PROGRAM P_Prog7
VAR

	fbKL6401 		: FB_LON_KL6401;

	fbREAD_191		: FB_READ_191_SNVT_log_status;
	fbSEND_191		: FB_SEND_191_SNVT_log_status;

	fbREAD_192		: FB_READ_192_SNVT_time_stamp_p;
	fbSEND_192		: FB_SEND_192_SNVT_time_stamp_p;

	fbREAD_193		: FB_READ_193_SNVT_log_fx_request;
	fbSEND_193		: FB_SEND_193_SNVT_log_fx_request;

	fbREAD_194		: FB_READ_194_SNVT_log_fx_status;
	fbSEND_194		: FB_SEND_194_SNVT_log_fx_status;

	fbREAD_195		: FB_READ_195_SNVT_log_request;
	fbSEND_195		: FB_SEND_195_SNVT_log_request;

	fbREAD_196		: FB_READ_196_SNVT_enthalpy_d;
	fbSEND_196		: FB_SEND_196_SNVT_enthalpy_d;

	fbREAD_197		: FB_READ_197_SNVT_amp_ac_mil;
	fbSEND_197		: FB_SEND_197_SNVT_amp_ac_mil;

	fbREAD_198		: FB_READ_198_SNVT_time_hour_p;
	fbSEND_198		: FB_SEND_198_SNVT_time_hour_p;

	fbREAD_199		: FB_READ_199_SNVT_lamp_status;
	fbSEND_199		: FB_SEND_199_SNVT_lamp_status;

	fbREAD_200		: FB_READ_200_SNVT_environment;
	fbSEND_200		: FB_SEND_200_SNVT_environment;

	fbREAD_201		: FB_READ_201_SNVT_geo_loc;
	fbSEND_201		: FB_SEND_201_SNVT_geo_loc;

END_VAR


fbKL6401(
	bDisabled:=FALSE ,
	stParameter_IN:=LON_IN_7 ,
	stParameter_OUT:=LON_OUT_7 ,
	stLON_Com:=stLON_Com_7,
	bReady=> ,
	eError=> ,
	stKL6401=> ,
	arrProgID=> ,
	arrNeuronID=> ,
	bBusy=> ,
	bError=> ,
	dwErrorKL=> ,
	bTimeOut=> ,
	byLONState=> );

(**)
fbREAD_191(
	wNVIndex:=0 ,
	bDisabled:= ,
	stLON_Com:=stLON_Com_7,
	stValue=> ,
	bNewData=> ,
	bError=> ,
	eError=> );
fbREAD_191.stValue;
fbREAD_191.bError;
fbREAD_191.eError;

fbSEND_191.stValue;
fbSEND_191.bStart;
fbSEND_191.bError;
fbSEND_191.eError;
fbSEND_191.bBusy;
fbSEND_191.dwErrorKL;

fbSEND_191.bAuto;
fbSEND_191.bSendInit;
fbSEND_191.tMinSendTime;
fbSEND_191.tMaxSendTime;

fbSEND_191(
	wNVIndex:=1 ,
	bStart:= ,
	stValue:= ,
	bDisabled:= ,
	stLON_Com:=stLON_Com_7,
	bError=> ,
	eError=> );
fbSEND_191.bStart:=FALSE;

(**)
fbREAD_192(
	wNVIndex:=2 ,
	bDisabled:= ,
	stLON_Com:=stLON_Com_7,
	stValue=> ,
	bNewData=> ,
	bError=> ,
	eError=> );
fbREAD_192.stValue;
fbREAD_192.bError;
fbREAD_192.eError;

fbSEND_192.stValue;
fbSEND_192.bStart;
fbSEND_192.bError;
fbSEND_192.eError;
fbSEND_192.bBusy;
fbSEND_192.dwErrorKL;

fbSEND_192.bAuto;
fbSEND_192.bSendInit;
fbSEND_192.tMinSendTime;
fbSEND_192.tMaxSendTime;

fbSEND_192(
	wNVIndex:=3 ,
	bStart:= ,
	stValue:= ,
	bDisabled:= ,
	stLON_Com:=stLON_Com_7,
	bError=> ,
	eError=> );
fbSEND_192.bStart:=FALSE;

(**)
fbREAD_193(
	wNVIndex:=4 ,
	bDisabled:= ,
	stLON_Com:=stLON_Com_7,
	stValue=> ,
	bNewData=> ,
	bError=> ,
	eError=> );
fbREAD_193.stValue;
fbREAD_193.bError;
fbREAD_193.eError;

fbSEND_193.stValue;
fbSEND_193.bStart;
fbSEND_193.bError;
fbSEND_193.eError;
fbSEND_193.bBusy;
fbSEND_193.dwErrorKL;

fbSEND_193.bAuto;
fbSEND_193.bSendInit;
fbSEND_193.tMinSendTime;
fbSEND_193.tMaxSendTime;

fbSEND_193(
	wNVIndex:=5 ,
	bStart:= ,
	stValue:= ,
	bDisabled:= ,
	stLON_Com:=stLON_Com_7,
	bError=> ,
	eError=> );
fbSEND_193.bStart:=FALSE;

(**)
fbREAD_194(
	wNVIndex:=6 ,
	bDisabled:= ,
	stLON_Com:=stLON_Com_7,
	stValue=> ,
	bNewData=> ,
	bError=> ,
	eError=> );
fbREAD_194.stValue;
fbREAD_194.bError;
fbREAD_194.eError;

fbSEND_194.stValue;
fbSEND_194.bStart;
fbSEND_194.bError;
fbSEND_194.eError;
fbSEND_194.bBusy;
fbSEND_194.dwErrorKL;

fbSEND_194.bAuto;
fbSEND_194.bSendInit;
fbSEND_194.tMinSendTime;
fbSEND_194.tMaxSendTime;

fbSEND_194(
	wNVIndex:=7 ,
	bStart:= ,
	stValue:= ,
	bDisabled:= ,
	stLON_Com:=stLON_Com_7,
	bError=> ,
	eError=> );
fbSEND_194.bStart:=FALSE;

(**)
fbREAD_195(
	wNVIndex:=8 ,
	bDisabled:= ,
	stLON_Com:=stLON_Com_7,
	uiValue=> ,
	bNewData=> ,
	bError=> ,
	eError=> );
fbREAD_195.uiValue;
fbREAD_195.bError;
fbREAD_195.eError;

fbSEND_195.uiValue;
fbSEND_195.bStart;
fbSEND_195.bError;
fbSEND_195.eError;
fbSEND_195.bBusy;
fbSEND_195.dwErrorKL;

fbSEND_195.bAuto;
fbSEND_195.bSendInit;
fbSEND_195.tMinSendTime;
fbSEND_195.tMaxSendTime;
fbSEND_195.uiValueLimit;

fbSEND_195(
	wNVIndex:=9 ,
	bStart:= ,
	uiValue:= ,
	bDisabled:= ,
	stLON_Com:=stLON_Com_7,
	bError=> ,
	eError=> );
fbSEND_195.bStart:=FALSE;

(**)
fbREAD_196(
	wNVIndex:=10 ,
	bDisabled:= ,
	stLON_Com:=stLON_Com_7,
	rValue=> ,
	bNewData=> ,
	bError=> ,
	eError=> );
fbREAD_196.rValue;
fbREAD_196.bError;
fbREAD_196.eError;

fbSEND_196.rValue;
fbSEND_196.bStart;
fbSEND_196.bError;
fbSEND_196.eError;
fbSEND_196.bBusy;
fbSEND_196.dwErrorKL;

fbSEND_196.bAuto;
fbSEND_196.bSendInit;
fbSEND_196.tMinSendTime;
fbSEND_196.tMaxSendTime;
fbSEND_196.rValueLimit;

fbSEND_196(
	wNVIndex:=11 ,
	bStart:= ,
	rValue:= ,
	bDisabled:= ,
	stLON_Com:=stLON_Com_7,
	bError=> ,
	eError=> );
fbSEND_196.bStart:=FALSE;

(**)
fbREAD_197(
	wNVIndex:=12 ,
	bDisabled:= ,
	stLON_Com:=stLON_Com_7,
	uiValue=> ,
	bNewData=> ,
	bError=> ,
	eError=> );
fbREAD_197.uiValue;
fbREAD_197.bError;
fbREAD_197.eError;

fbSEND_197.uiValue;
fbSEND_197.bStart;
fbSEND_197.bError;
fbSEND_197.eError;
fbSEND_197.bBusy;
fbSEND_197.dwErrorKL;

fbSEND_197.bAuto;
fbSEND_197.bSendInit;
fbSEND_197.tMinSendTime;
fbSEND_197.tMaxSendTime;
fbSEND_197.uiValueLimit;

fbSEND_197(
	wNVIndex:=13 ,
	bStart:= ,
	uiValue:= ,
	bDisabled:= ,
	stLON_Com:=stLON_Com_7,
	bError=> ,
	eError=> );
fbSEND_197.bStart:=FALSE;

(**)
fbREAD_198(
	wNVIndex:=14 ,
	bDisabled:= ,
	stLON_Com:=stLON_Com_7,
	udiValue=> ,
	bNewData=> ,
	bError=> ,
	eError=> );
fbREAD_198.udiValue;
fbREAD_198.bError;
fbREAD_198.eError;

fbSEND_198.udiValue;
fbSEND_198.bStart;
fbSEND_198.bError;
fbSEND_198.eError;
fbSEND_198.bBusy;
fbSEND_198.dwErrorKL;

fbSEND_198.bAuto;
fbSEND_198.bSendInit;
fbSEND_198.tMinSendTime;
fbSEND_198.tMaxSendTime;
fbSEND_198.udiValueLimit;

fbSEND_198(
	wNVIndex:=15 ,
	bStart:= ,
	udiValue:= ,
	bDisabled:= ,
	stLON_Com:=stLON_Com_7,
	bError=> ,
	eError=> );
fbSEND_198.bStart:=FALSE;

(**)
fbREAD_199(
	wNVIndex:=16 ,
	bDisabled:= ,
	stLON_Com:=stLON_Com_7,
	stValue=> ,
	bNewData=> ,
	bError=> ,
	eError=> );
fbREAD_199.stValue;
fbREAD_199.bError;
fbREAD_199.eError;

fbSEND_199.stValue;
fbSEND_199.bStart;
fbSEND_199.bError;
fbSEND_199.eError;
fbSEND_199.bBusy;
fbSEND_199.dwErrorKL;

fbSEND_199.bAuto;
fbSEND_199.bSendInit;
fbSEND_199.tMinSendTime;
fbSEND_199.tMaxSendTime;

fbSEND_199(
	wNVIndex:=17 ,
	bStart:= ,
	stValue:= ,
	bDisabled:= ,
	stLON_Com:=stLON_Com_7,
	bError=> ,
	eError=> );
fbSEND_199.bStart:=FALSE;

(**)
fbREAD_200(
	wNVIndex:=18 ,
	bDisabled:= ,
	stLON_Com:=stLON_Com_7,
	stValue=> ,
	bNewData=> ,
	bError=> ,
	eError=> );
fbREAD_200.stValue;
fbREAD_200.bError;
fbREAD_200.eError;

fbSEND_200.stValue;
fbSEND_200.bStart;
fbSEND_200.bError;
fbSEND_200.eError;
fbSEND_200.bBusy;
fbSEND_200.dwErrorKL;

fbSEND_200.bAuto;
fbSEND_200.bSendInit;
fbSEND_200.tMinSendTime;
fbSEND_200.tMaxSendTime;

fbSEND_200(
	wNVIndex:=19 ,
	bStart:= ,
	stValue:= ,
	bDisabled:= ,
	stLON_Com:=stLON_Com_7,
	bError=> ,
	eError=> );
fbSEND_200.bStart:=FALSE;

(**)
fbREAD_201(
	wNVIndex:=20 ,
	bDisabled:= ,
	stLON_Com:=stLON_Com_7,
	stValue=> ,
	bNewData=> ,
	bError=> ,
	eError=> );
fbREAD_201.stValue;
fbREAD_201.bError;
fbREAD_201.eError;

fbSEND_201.stValue;
fbSEND_201.bStart;
fbSEND_201.bError;
fbSEND_201.eError;
fbSEND_201.bBusy;
fbSEND_201.dwErrorKL;

fbSEND_201.bAuto;
fbSEND_201.bSendInit;
fbSEND_201.tMinSendTime;
fbSEND_201.tMaxSendTime;

fbSEND_201(
	wNVIndex:=21 ,
	bStart:= ,
	stValue:= ,
	bDisabled:= ,
	stLON_Com:=stLON_Com_7,
	bError=> ,
	eError=> );
fbSEND_201.bStart:=FALSE;

END_PROGRAM
